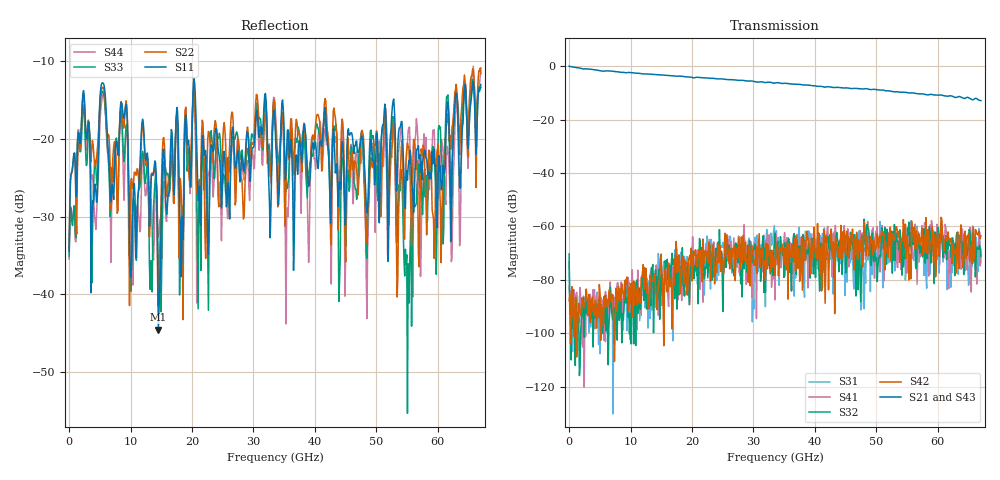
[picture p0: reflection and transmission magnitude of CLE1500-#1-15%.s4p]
!Keysight Technologies,N5247B,US50470101,A.16.20.02
!Date: Thursday, March 13, 2025 10:11:58
!Correction: S11(C  4-Port  )
!S12(C  4-Port  )
!S13(C  4-Port  )
!S14(C  4-Port  )
!S21(C  4-Port  )
!S22(C  4-Port  )
!S23(C  4-Port  )
!S24(C  4-Port  )
!S31(C  4-Port  )
!S32(C  4-Port  )
!S33(C  4-Port  )
!S34(C  4-Port  )
!S41(C  4-Port  )
!S42(C  4-Port  )
!S43(C  4-Port  )
!S44(C  4-Port  )
!S4P File: Measurements: <S11,S12,S13,S14>,
!<S21,S22,S23,S24>,
!<S31,S32,S33,S34>,
!<S41,S42,S43,S44>:
# Hz S  dB  R 50
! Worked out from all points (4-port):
!   601 points, 10 MHz to 67 GHz, reference 50 ohm
!   strongest paths, dB at 10 MHz, 16.76 GHz, 33.51 GHz, 50.25 GHz, 67 GHz:
!     S21: 0.0, -3.6, -6.3, -8.9, -12.9
!     S43: 0.0, -3.6, -6.4, -9.0, -12.6
!     S42: -87.9, -98.4, -78.4, -66.3, -63.5
!     S32: -70.3, -70.2, -62.5, -75.0, -71.3
!     S41: -82.5, -76.2, -87.6, -74.1, -68.6
!     S31: -73.2, -70.1, -63.8, -64.8, -73.6
!   lowest |S11| = -44.6 dB at 14.52 GHz (marker M1), VSWR 1.01, Z = 50.5 - j0.328 ohm
!   |S11| at or under -10 dB: start of sweep to end of sweep
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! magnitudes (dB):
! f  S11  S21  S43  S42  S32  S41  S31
! 10 MHz  -34.5  0.0  0.0  -87.9  -70.3  -82.5  -73.2
! 5.481 GHz  -12.8  -1.9  -1.7  -90.5  -100.2  -95.8  -91.7
! 14.52 GHz  -44.6  -3.2  -3.1  -82.9  -87.1  -93.3  -70.2
! 20.33 GHz  -12.3  -4.4  -4.3  -69.6  -79.7  -75.7  -79.3
! 51.15 GHz  -18.2  -9.0  -9.0  -62.4  -68.2  -70.2  -72.2
! 55.39 GHz  -23.2  -10.0  -10.5  -70.6  -60.4  -69.1  -68.8
! 67 GHz  -13.0  -12.9  -12.6  -63.5  -71.3  -68.6  -73.6
